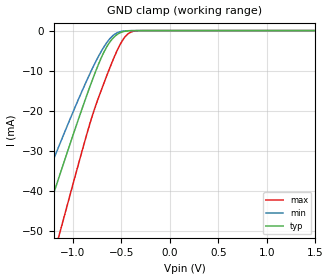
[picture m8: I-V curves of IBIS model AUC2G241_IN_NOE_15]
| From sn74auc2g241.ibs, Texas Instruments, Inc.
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[Model]   AUC2G241_IN_NOE_15
Model_type  Input
Vinl=0.49
Vinh=1.04
| variable   typ   min   max
C_comp   2.62pF   2.19pF   3.01pF
[Temperature Range]   40   100   -40
| Ambient temperature   25   85   -40
[Voltage range]   1.5   1.4   1.6
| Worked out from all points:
|   GND clamp passes 1 mA (typ) near -0.55 V on its own axis
[GND Clamp]
| AUC2G241_IN_NOE_15
|   Voltage   I(typ)   I(min)   I(max)
-3.6V     -223.1mA   -186.8mA   -268.3mA
-1.505V   -63.61mA   -50.93mA   -83.59mA
-1.46V    -60.22mA   -48.13mA   -79.57mA
-1.325V   -50.08mA   -39.79mA   -67.5mA
-1.17V    -38.57mA   -30.39mA   -53.61mA
-1.12V    -34.89mA   -27.41mA   -49.13mA
-840mV    -15.01mA   -11.55mA   -24.46mA
-695mV    -6.121mA   -4.657mA   -14.06mA
-570mV    -1.488mA   -922uA     -6.381mA
-430mV    -73.19uA   -35.15uA   -776.9uA
-280mV    -781.4nA   -560.5nA   -5.358uA
1.5V      174.7pA    268pA      181.1pA
